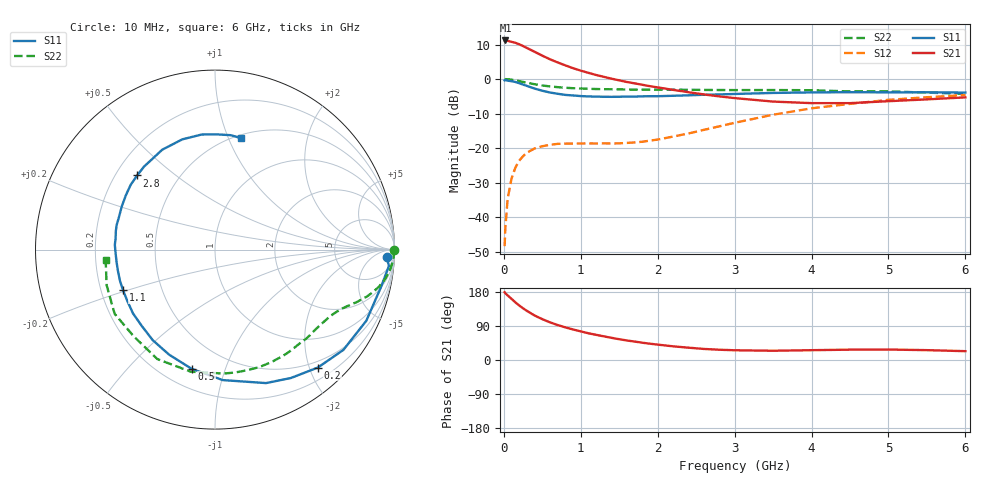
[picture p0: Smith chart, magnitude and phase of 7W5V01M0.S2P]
! Infineon Technologies  Discrete & RF Semiconductors
! BFS17W
! Si NPN RF Bipolar Junction Transistor in SOT323
! VCE = 5 V  IC = 1 mA
! Common Emitter S-Parameters:  August  1999
# GHz  S  MA  R  50
!  f  S11  S21  S12  S22
! GHz  MAG  ANG  MAG  ANG  MAG  ANG  MAG  ANG
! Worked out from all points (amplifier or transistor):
!   36 points, 10 MHz to 6 GHz, reference 50 ohm
!   highest |S21| = 11.2 dB at 20 MHz (marker M1)
!   |S21| within 3 dB of that: start of sweep to 374.5 MHz
!   unconditionally stable (mu >= 1): 1.053 GHz to end of sweep
!   at 250 MHz: K = 0.26, MSG = 15.9 dB, |S12| = -22.3 dB
!   at 1.4 GHz: K = 1.25, MAG = 6.4 dB, |S12| = -18.7 dB
!   at 6 GHz: K = 1.09, MAG = -2.2 dB, |S12| = -4.6 dB
!   S11 on the Smith chart (normalised r, x): 10 MHz: 23, -23; 200 MHz: 0.39, -2.14; 500 MHz: 0.32, -0.77; 1.1 GHz: 0.29, -0.19; 2.8 GHz: 0.29, +0.37; 6 GHz: 0.53, +1.11
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0.01  0.9573 -2.5  3.591 178.8  0.0038 82.9  0.9999 -0.2
0.02  0.9735 -5.4  3.623 176.2  0.0071 88.1  0.9971 -1.4
0.05  0.9476 -12.9  3.576 170.3  0.0186 84.0  0.9937 -3.7
0.1  0.9316 -25.2  3.46 161.4  0.0363 76.3  0.9798 -7.1
0.15  0.9077 -38.0  3.352 152.1  0.0523 68.2  0.9584 -10.3
0.2  0.8719 -48.9  3.189 143.9  0.0656 63.1  0.9349 -12.9
0.25  0.8311 -59.4  3.009 136.4  0.0765 57.0  0.9085 -15.3
0.3  0.7961 -69.1  2.817 129.6  0.0859 52.8  0.8853 -17.2
0.4  0.7283 -86.6  2.484 117.4  0.0988 45.6  0.8412 -20.4
0.5  0.6772 -101.0  2.182 107.8  0.1064 40.5  0.8072 -22.7
0.6  0.6387 -113.6  1.934 99.3  0.1117 37.2  0.7824 -24.7
0.7  0.6123 -124.5  1.741 92.3  0.1152 35.0  0.7636 -26.8
0.9  0.5789 -142.1  1.437 80.5  0.1164 32.6  0.7375 -30.9
1.1  0.5603 -156.3  1.23 70.5  0.117 33.2  0.7227 -35.1
1.6  0.5587 177.3  0.906 51.5  0.1189 42.2  0.7052 -47.1
2.2  0.5725 155.1  0.698 36.1  0.1468 58.6  0.7011 -63.3
2.8  0.599 136.4  0.561 27.1  0.2066 66.3  0.6939 -80.7
3.5  0.6295 117.8  0.472 24.4  0.3045 64.8  0.6934 -101.3
4.5  0.6455 96.6  0.448 27.3  0.4373 52.5  0.6622 -133.3
5  0.642 88.9  0.478 27.6  0.4998 45.8  0.6638 -147.4
5.5  0.6435 82.1  0.508 26.0  0.5456 39.0  0.6356 -161.8
6  0.6373 76.8  0.543 23.3  0.5859 32.6  0.612 -174.4
